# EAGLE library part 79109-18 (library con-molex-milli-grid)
RECEPTACAL
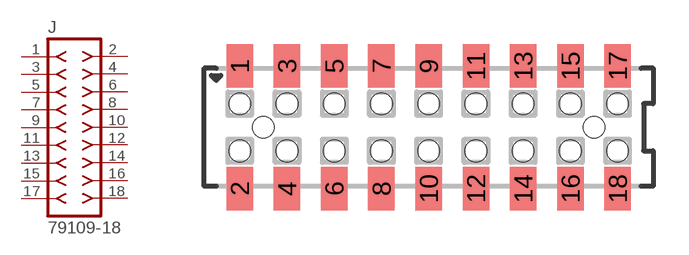
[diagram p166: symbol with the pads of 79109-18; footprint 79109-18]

Designator prefix J

## 79109-18  [79109-18]
1  1  pas
2  2  pas
3  3  pas
4  4  pas
5  5  pas
6  6  pas
7  7  pas
8  8  pas
9  9  pas
10  10  pas
11  11  pas
12  12  pas
13  13  pas
14  14  pas
15  15  pas
16  16  pas
17  17  pas
18  18  pas

## Footprint 79109-18 (pad centres in mm)
RECEPTACAL SMD Dual Row, Vertical, Pass-Thru
smd 1.12 x 1.83: 1 -8,2.6; 2 -8,-2.6; 3 -6,2.6; 4 -6,-2.6; 5 -4,2.6; 6 -4,-2.6; 7 -2,2.6; 8 -2,-2.6; 9 0,2.6; 10 0,-2.6; 11 2,2.6; 12 2,-2.6; 13 4,2.6; 14 4,-2.6; 15 6,2.6; 16 6,-2.6; 17 8,2.6; 18 8,-2.6
hole 0.914 at -7,0
hole 0.914 at -8,1
hole 0.914 at -8,-1
hole 0.914 at -6,-1
hole 0.914 at -6,1
hole 0.914 at -4,-1
hole 0.914 at -4,1
hole 0.914 at 7,0
hole 0.914 at -2,1
hole 0.914 at -2,-1
hole 0.914 at 0,1
hole 0.914 at 0,-1
hole 0.914 at 2,1
hole 0.914 at 2,-1
hole 0.914 at 4,1
hole 0.914 at 4,-1
hole 0.914 at 6,-1
hole 0.914 at 6,1
hole 0.914 at 8,1
hole 0.914 at 8,-1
